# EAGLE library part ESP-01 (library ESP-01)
Check availability
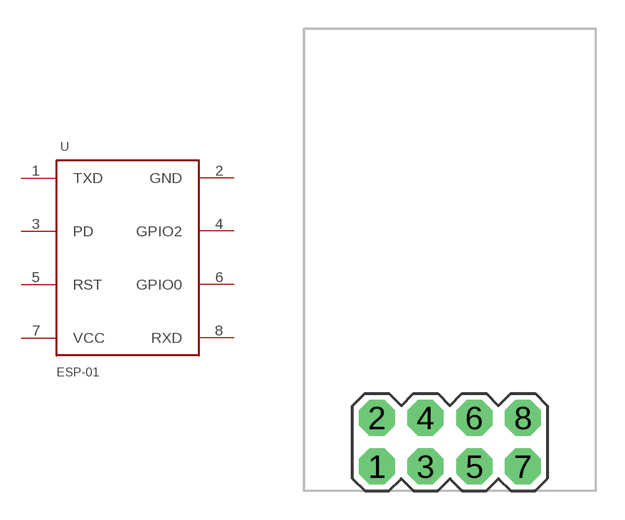
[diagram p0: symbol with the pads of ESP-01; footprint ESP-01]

Designator prefix -

## ESP-01 (Availability: Not in stock; Description: ESP-01M ESP8266 DIP Adapter series Transceiver; 802.11 b/g/n (Wi-Fi, WiFi, WLAN) Evaluation Board; MF: AI-Thinker; MP: ESP-01; Package: Non-Standard AI-Thinker; Price: None)  [ESP-01]
1  TXD
2  GND
3  PD
4  GPIO2
5  RST
6  GPIO0
7  VCC
8  RXD

## Footprint ESP-01 (pad centres in mm)
drill 1.016 pad 1.88 octagon: 1 -3.81,-1.27; 2 -3.81,1.27; 3 -1.27,-1.27; 4 -1.27,1.27; 5 1.27,-1.27; 6 1.27,1.27; 7 3.81,-1.27; 8 3.81,1.27

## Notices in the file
This work is licensed under a Creative Commons Attribution-ShareAlike 4.0 International License (CC BY-SA) with Design Exception 1.0
